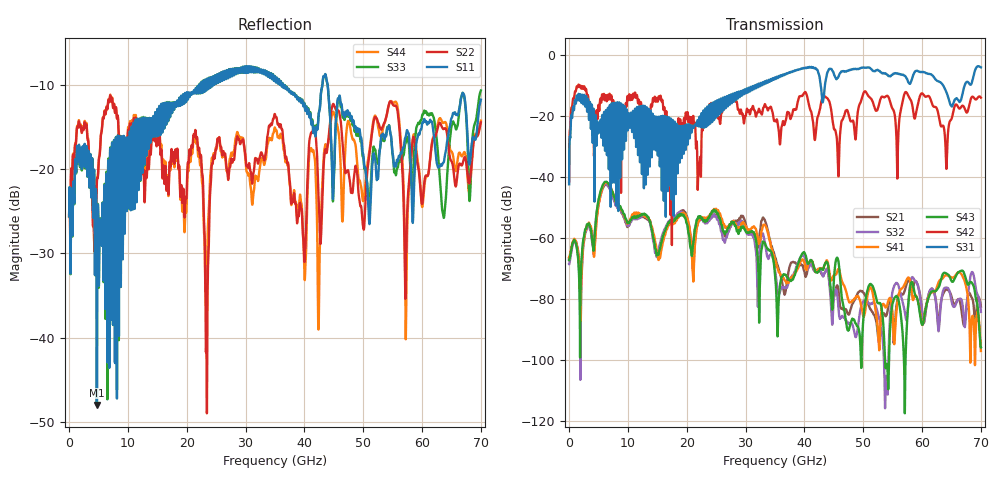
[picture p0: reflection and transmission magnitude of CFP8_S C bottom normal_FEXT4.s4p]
! AWR Design Environment (8415) Tue Jan 08 14:03:21 2019
! Document = 'CFP8 Channel_S_2'
! nPorts: 4, nXvals: 7001
# HZ S DB R 50
!Freq DBS11 AngS11 DBS12 AngS12 DBS13 AngS13 DBS14 AngS14
!	DBS21 AngS21 DBS22 AngS22 DBS23 AngS23 DBS24 AngS24
!	DBS31 AngS31 DBS32 AngS32 DBS33 AngS33 DBS34 AngS34
!	DBS41 AngS41 DBS42 AngS42 DBS43 AngS43 DBS44 AngS44
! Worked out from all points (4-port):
!   7000 points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, 10 MHz to 70 GHz, reference 50 ohm
!   strongest paths, dB at 10 MHz, 17.51 GHz, 35.01 GHz, 52.51 GHz, 70 GHz:
!     S31: -42.4, -26.3, -7.5, -4.9, -4.0
!     S42: -41.6, -38.6, -21.6, -17.4, -14.0
!     S43: -67.3, -54.3, -72.0, -81.4, -96.0
!     S41: -66.5, -55.0, -67.3, -90.0, -97.1
!     S32: -68.6, -53.8, -70.5, -85.1, -84.3
!     S21: -66.9, -54.5, -66.3, -92.1, -82.5
!   lowest |S11| = -48.0 dB at 4.73 GHz (marker M1), VSWR 1.01, Z = 49.9 - j0.396 ohm
!   |S11| at or under -10 dB: start of sweep to 22.16 GHz; 36.38 GHz to 43.05 GHz (6.671 GHz wide, 16.8 % of centre); 43.96 GHz to end of sweep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
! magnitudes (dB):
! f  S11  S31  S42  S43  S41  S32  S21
! 10 MHz  -25.6  -42.4  -41.6  -67.3  -66.5  -68.6  -66.9
! 1.35 GHz  -17.4  -13.4  -10.3  -63.7  -62.8  -63.6  -62.5
! 4.73 GHz  -48.0  -23.0  -18.9  -51.0  -53.2  -51.0  -52.9
! 22.12 GHz  -10.3  -21.0  -36.3  -53.3  -54.3  -53.4  -54.4
! 23.42 GHz  -9.8  -18.5  -19.2  -54.4  -53.5  -55.1  -54.3
! 27.24 GHz  -8.3  -14.5  -13.7  -56.0  -56.0  -56.8  -57.0
! 70 GHz  -11.8  -4.0  -14.0  -96.0  -97.1  -84.3  -82.5
